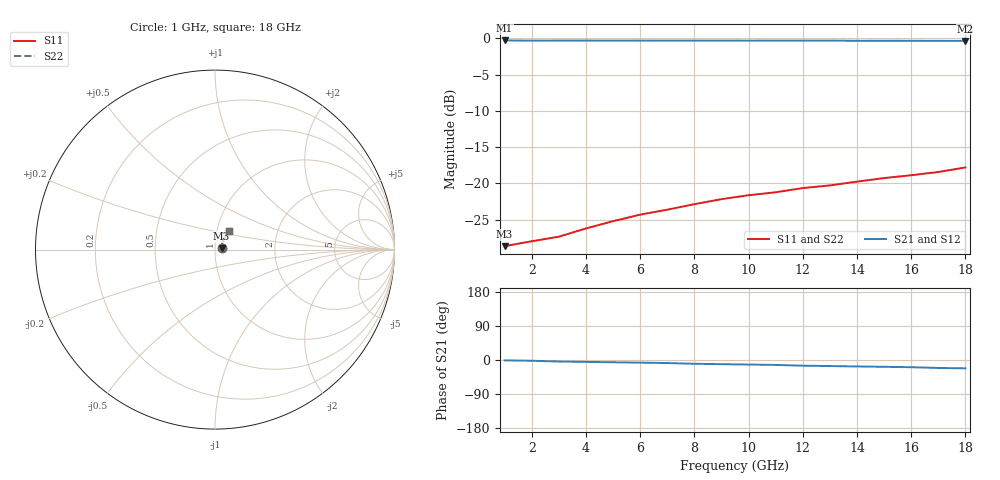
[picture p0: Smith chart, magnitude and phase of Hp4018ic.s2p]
!HPND-4018 beam lead PIN diode
!Series configuration S-parameters If=10mA.  Last updated 10/3/97
# mhz s ma r 50
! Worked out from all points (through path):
!   18 points, 1 GHz to 18 GHz, reference 50 ohm
!   highest |S21| = -0.29 dB at 1 GHz (marker M1); lowest = -0.4 dB at 18 GHz (marker M2)
!   group delay of S21, straight-line fit = 3.4 ps
!   lowest |S11| = -28.6 dB at 1 GHz (marker M3), VSWR 1.08, Z = 53.8 + j0.76 ohm
!   |S11| at or under -10 dB: start of sweep to end of sweep
!   |S22| runs from -28.6 to -17.8 dB; largest |S21 - S12| = 0
1000  0.037 11.0  0.967 -1.0  0.967 -1.0  0.037 11.0
2000  0.04 23.0  0.965 -2.0  0.965 -2.0  0.04 23.0
3000  0.043 32.0  0.966 -4.0  0.966 -4.0  0.043 32.0
4000  0.049 38.0  0.966 -5.0  0.966 -5.0  0.049 38.0
5000  0.055 43.0  0.965 -6.0  0.965 -6.0  0.055 43.0
6000  0.061 46.0  0.965 -7.0  0.965 -7.0  0.061 46.0
7000  0.066 48.0  0.965 -8.0  0.965 -8.0  0.066 48.0
8000  0.072 50.0  0.965 -10.0  0.965 -10.0  0.072 50.0
9000  0.078 51.0  0.965 -11.0  0.965 -11.0  0.078 51.0
10000  0.083 51.0  0.964 -12.0  0.964 -12.0  0.083 51.0
11000  0.087 52.0  0.965 -13.0  0.965 -13.0  0.087 52.0
12000  0.093 52.0  0.965 -15.0  0.965 -15.0  0.093 52.0
13000  0.097 52.0  0.965 -16.0  0.965 -16.0  0.097 52.0
14000  0.103 53.0  0.962 -17.0  0.962 -17.0  0.103 53.0
15000  0.109 53.0  0.963 -18.0  0.963 -18.0  0.109 53.0
16000  0.114 53.0  0.962 -19.0  0.962 -19.0  0.114 53.0
17000  0.12 53.0  0.961 -21.0  0.961 -21.0  0.12 53.0
18000  0.129 53.0  0.96 -22.0  0.96 -22.0  0.129 53.0
